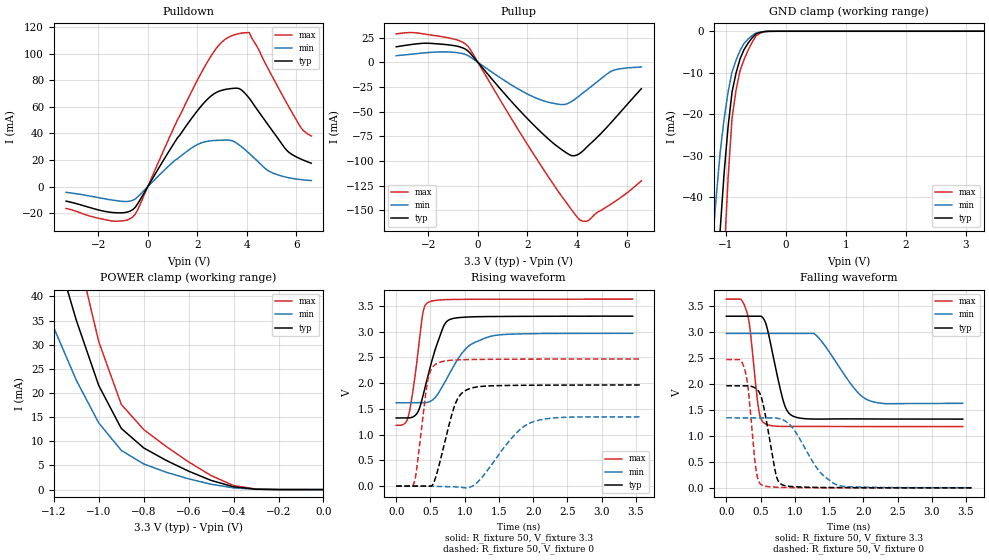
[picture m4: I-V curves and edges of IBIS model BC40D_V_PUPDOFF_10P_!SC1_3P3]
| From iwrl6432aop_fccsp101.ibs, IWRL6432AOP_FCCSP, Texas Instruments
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|   Model Cell BC40D_V_PUPDOFF_10P_!SC1_3P3
|BC40D_V_PUPDOFF_10P_!SC1_3P3
[Model]   BC40D_V_PUPDOFF_10P_!SC1_3P3
Model_type   I/O
Polarity   Non-Inverting
Enable   Active-Low
Vinl =  0.8V
Vinh =  2V
Cref =  15pF
Rref =  100.0000M
Vref =  0V
Vmeas =  1.65
C_comp   2.059994p   1.912853p   2.135747p
|[Input load] weak_pupdoff
|[Output drive] fast
|[supplytol] 10
|[temp] ind
[Model Spec]
Vinl   0.8V   0.8V   0.8V
Vinh   2V   2V   2V
[Temperature Range]   25   125   -40
[Voltage Range]   3.3   2.97   3.63
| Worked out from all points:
|   slope of the pulldown table from 0 to 0.495 V, typ, clamps not added: 31.8 ohm
|   slope of the pullup table from 0 to 0.495 V, typ, clamps not added: 33.3 ohm
|   GND clamp passes 1 mA (typ) near -0.53 V on its own axis
|   POWER clamp passes 1 mA (typ) near -0.43 V on its own axis
|   rising waveform, R_fixture 50, V_fixture 3.3: 20-80 % time 251ps typ, 385ps min, 143ps max; typ from 1.32 V to 3.3 V
|   rising waveform, R_fixture 50, V_fixture 0: 20-80 % time 232ps typ, 477ps min, 136ps max; typ from 0 V to 1.96 V
|   falling waveform, R_fixture 50, V_fixture 3.3: 20-80 % time 196ps typ, 423ps min, 118ps max; typ from 3.3 V to 1.32 V
|   falling waveform, R_fixture 50, V_fixture 0: 20-80 % time 160ps typ, 381ps min, 106ps max; typ from 1.96 V to 0 V
| Nom Voltages:
|   VDD=1.1001, VDDS=3.3, VDDS18=1.8, ESD_BIASFET=0, VSS=0, VSSS=0
| Min Voltages:
|   VDD=0.99, VDDS=2.97, VDDS18=1.62, ESD_BIASFET=0, VSS=0, VSSS=0
| Max Voltages:
|   VDD=1.21, VDDS=3.63, VDDS18=1.98, ESD_BIASFET=0, VSS=0, VSSS=0
[POWER_clamp]
|   voltage   I(typ)   I(min)   I(max)
-3.3V     446.9mA    419.5mA    603.9mA
-1.267V   62.17mA    41.5mA     88.03mA
-1.233V   56.52mA    37.5mA     80.22mA
-1.133V   40.34mA    26.27mA    57.61mA
-1.067V   30.56mA    19.7mA     43.68mA
-1.033V   26.05mA    16.75mA    37.15mA
-1V       21.55mA    13.8mA     30.62mA
-900mV    12.68mA    8.135mA    17.65mA
-800mV    8.63mA     5.309mA    12.43mA
-600mV    3.813mA    2.231mA    5.733mA
-400mV    580.7uA    357.1uA    842.6uA
0V        4.589uA    2.01uA     9.301uA
[Pulldown]
|   voltage   I(typ)   I(min)   I(max)
-3.3V     -10.92mA   -4.307mA   -16.45mA
-1.4V     -19.52mA   -10.22mA   -25.94mA
-600mV    -17.22mA   -10.25mA   -22.66mA
1.1V      33.8mA     19.88mA    46.22mA
2.1V      59.3mA     32.44mA    83.48mA
2.9V      71.86mA    34.84mA    107mA
3.5V      73.95mA    33.66mA    114.2mA
4.1V      66.34mA    24.89mA    115.8mA
4.9V      45.33mA    11.53mA    87.2mA
5.6V      27.47mA    7.046mA    63.1mA
6.2V      20.56mA    5.221mA    43.87mA
6.6V      17.6mA     4.555mA    38.05mA
[Pullup]
|   voltage   I(typ)   I(min)   I(max)
-3.3V     15.77mA    6.741mA    28.8mA
-1.9V     19.23mA    10.15mA    27.67mA
-900mV    16.69mA    10.02mA    23.17mA
-400mV    11.53mA    6.853mA    16.25mA
1.3V      -38.16mA   -22.04mA   -54.89mA
2.3V      -64.7mA    -35.66mA   -95.04mA
3.4V      -88.76mA   -42.82mA   -136.4mA
3.8V      -94.64mA   -39.36mA   -150mA
4.1V      -92.52mA   -33.79mA   -159.3mA
4.4V      -85.77mA   -27.94mA   -161mA
5.4V      -60.46mA   -8.849mA   -143.2mA
6.6V      -26.71mA   -4.741mA   -120mA
[GND_clamp]
|   voltage   I(typ)   I(min)   I(max)
-3.3V     -787.2mA   -607.8mA   -1.235A
-1.233V   -85.66mA   -52.14mA   -138.8mA
-1.167V   -66.47mA   -40.37mA   -107.7mA
-1.1V     -48.25mA   -29.37mA   -77.98mA
-1.033V   -34.27mA   -21.19mA   -54.56mA
-966.7mV  -23.06mA   -14.66mA   -35.51mA
-900mV    -14.61mA   -9.789mA   -20.83mA
-833.3mV  -10.05mA   -6.934mA   -14.15mA
-700mV    -4.416mA   -2.931mA   -6.81mA
-500mV    -621.6uA   -443.4uA   -1.094mA
-300mV    -17.13uA   -24.29uA   -23.57uA
3.3V      4.589uA    110.6uA    5.608uA
[Ramp]
| variable   typ   min   max
dV/dt_f  1.1959433/0.19777536n 0.83580782/0.43959778n  1.4762235/0.11853739n
dV/dt_r  1.1917531/0.2345539n 0.82901977/0.48916151n  1.4908433/0.13717949n
R_load = 50
[Rising Waveform]
R_fixture = 50
V_fixture = 3.3
V_fixture_min = 2.97
V_fixture_max = 3.63
|   time   V(typ)   V(min)   V(max)
0s        1.322V     1.617V     1.18V
178.4ps   1.322V     1.617V     1.36V
305.5ps   1.415V     1.617V     2.455V
387.2ps   1.732V     1.617V     3.341V
470.7ps   2.178V     1.631V     3.569V
684.6ps   3.081V     1.957V     3.618V
811.7ps   3.248V     2.264V     3.623V
1.057ns   3.283V     2.716V     3.626V
1.417ns   3.292V     2.919V     3.628V
3.453ns   3.299V     2.966V     3.63V
[Rising Waveform]
R_fixture = 50
V_fixture = 0
V_fixture_min = 0
V_fixture_max = 0
|   time   V(typ)   V(min)   V(max)
0s        0V         0V         0V
261.9ps   0V         0V         65.75mV
296.9ps   0V         0V         308.5mV
461.7ps   0V         0V         2.052V
529.1ps   19.27mV    -3.671mV   2.304V
597.6ps   264.7mV    -5.417mV   2.381V
855ps     1.568V     -14.09mV   2.448V
1.045ns   1.877V     -30.97mV   2.456V
1.973ns   1.958V     1.235V     2.465V
3.581ns   1.963V     1.344V     2.468V
[Falling Waveform]
R_fixture = 50
V_fixture = 3.3
V_fixture_min = 2.97
V_fixture_max = 3.63
|   time   V(typ)   V(min)   V(max)
0s        3.301V     2.97V      3.629V
295.6ps   3.301V     2.97V      3.399V
346.7ps   3.301V     2.97V      3.046V
475.6ps   3.301V     2.97V      1.483V
569.4ps   3.187V     2.97V      1.232V
833.3ps   1.664V     2.97V      1.181V
967.5ps   1.383V     2.97V      1.181V
1.307ns   1.322V     2.939V     1.181V
2.078ns   1.325V     1.683V     1.179V
3.453ns   1.322V     1.626V     1.179V
[Falling Waveform]
R_fixture = 50
V_fixture = 0
V_fixture_min = 0
V_fixture_max = 0
|   time   V(typ)   V(min)   V(max)
0s        1.963V     1.347V     2.467V
271.3ps   1.962V     1.347V     2.264V
320.4ps   1.961V     1.347V     1.889V
430ps     1.912V     1.347V     377.8mV
520ps     1.702V     1.347V     52.95mV
722.5ps   270.5mV    1.343V     12.4mV
820.1ps   56.2mV     1.31V      7.54mV
1.352ns   8.197mV    328.6mV    0V
1.621ns   5.571mV    54.71mV    0V
3.581ns   0V         3.118mV    0V
